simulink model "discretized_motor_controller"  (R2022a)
settings: Solver=VariableStepAuto  StartTime=0.0  StopTime=10  RelTol=1e-3
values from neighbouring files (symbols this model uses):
  B = 1e-5    (= 1e-05)    [motor_controller.m]
  J = 1e-4    (= 0.0001)    [motor_controller.m]
  k = 2e-2    (= 0.02)    [motor_controller.m]
  Ka_i = 1 / Kp_i    (= 0.2)    [motor_controller.m]
  Ka_s = 1 / Kp_s    (= 0.2)    [motor_controller.m]
  Ki_i = Kp_i * Ra / La    (= 1000)    [motor_controller.m]
  Ki_s = J * omega_cs^2 / (5 * k)    (= 1000)    [motor_controller.m]
  Kp_i = La * omega_cc    (= 5)    [motor_controller.m]
  Kp_p = 2.5    [motor_controller.m]
  Kp_s = J * omega_cs / k    (= 5)    [motor_controller.m]
  La = 1e-3    (= 0.001)    [motor_controller.m]
  Ra = 0.2    [motor_controller.m]
  T_sample = 1 / f_sample    (= 1e-05)    [motor_controller.m]
undefined symbols (not defined in the file or in its folder): DiscIntNeverNeededParam

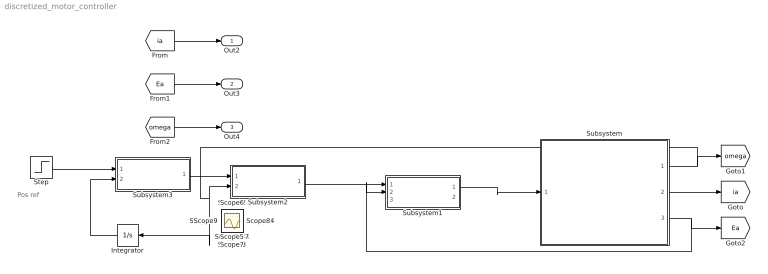
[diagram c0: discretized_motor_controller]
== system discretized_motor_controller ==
  note: Pos ref
  Integrator : Integrator
  Step : Step  After=180  SampleTime=0
  Subsystem : Subsystem  Tag=PMDC  Description=PMDC
  Subsystem1 : Subsystem  Description=PI controller
  Subsystem2 : Subsystem  Description=PI controller
  Subsystem3 : Subsystem  Description=PI controller
  Out2 : Outport
  Out3 : Outport  Port=2
  Out4 : Outport  Port=3
  Scope{,1..34} (35 alike) : Scope
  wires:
  Subsystem/1(Out1) -> Subsystem2/2(In4), Integrator/1, [omega]
  [ia] -> Out2/1
  [Ea] -> Out3/1
  [omega] -> Out4/1
  Subsystem/3(Out3) -> Subsystem1/2(In2), [Ea]
  Subsystem/2(Out2) -> [ia]
  Step/1 -> Subsystem3/1(In1)
  Integrator/1 -> Subsystem3/2(In3)
  Subsystem3/1(Out1) -> Subsystem2/1(In1)
  Subsystem1/1(Out1) -> Subsystem/1(In1)
  Subsystem2/1(Out2) -> Subsystem1/1(In1)

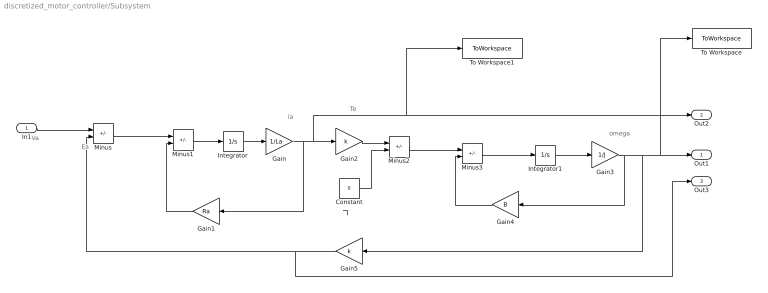
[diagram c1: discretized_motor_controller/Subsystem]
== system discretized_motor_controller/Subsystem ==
  note: Ea
  note: Va
  note: Te
  note: Tl
  note: omega
  note: ia
  In1 : Inport
  Constant : Constant  Value=0
  Gain : Gain  Gain=1/La
  Gain1 : Gain  Gain=Ra
  Gain2 : Gain  Gain=k
  Gain3 : Gain  Gain=1/J
  Gain4 : Gain  Gain=B
  Gain5 : Gain  Gain=k
  Integrator : Integrator
  Integrator1 : Integrator
  Minus{,1..3} (4 alike) : Sum  Inputs=+-
  To Workspace : ToWorkspace  VariableName=omega_simout  SaveFormat=Timeseries  SampleTime=-1
  To Workspace1 : ToWorkspace  VariableName=current_simout  SaveFormat=Timeseries  SampleTime=-1
  Out1 : Outport
  Out2 : Outport  Port=2
  Out3 : Outport  Port=3
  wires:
  Minus/1 -> Minus1/1
  Gain1/1 -> Minus1/2
  Minus1/1 -> Integrator/1
  Integrator/1 -> Gain/1
  Gain/1 -> To Workspace1/1, Out2/1, Gain2/1, Gain1/1
  Gain2/1 -> Minus2/1
  Constant/1 -> Minus2/2
  Minus2/1 -> Minus3/1
  Minus3/1 -> Integrator1/1
  Integrator1/1 -> Gain3/1
  Gain4/1 -> Minus3/2
  In1/1 -> Minus/1
  Gain5/1 -> Out3/1, Minus/2
  Gain3/1 -> Gain4/1, Gain5/1, To Workspace/1, Out1/1

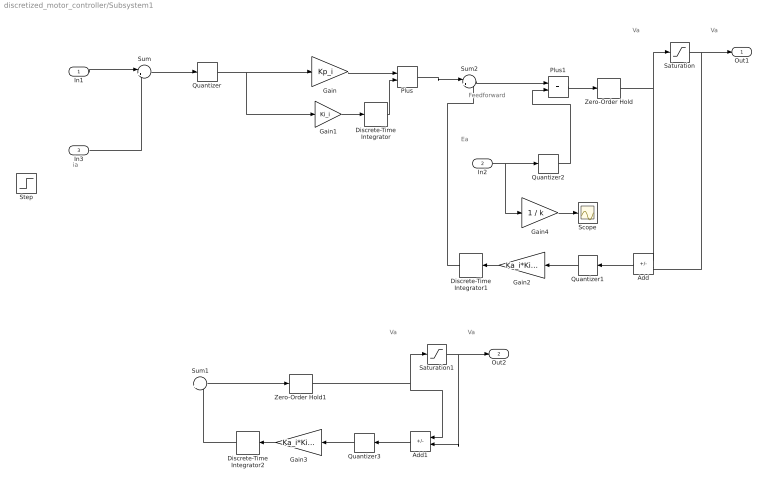
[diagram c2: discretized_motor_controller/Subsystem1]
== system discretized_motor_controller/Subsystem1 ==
  note: ia
  note: Ea
  note: Feedforward
  note: Va
  note: Va
  note: Va
  note: Va
  In1 : Inport
  In2 : Inport  Port=2
  In3 : Inport  Port=3
  Add : Sum  Inputs=+-
  Add1 : Sum  Inputs=+-
  Discrete-Time Integrator : DiscreteIntegrator  SampleTime=T_sample  ICPrevOutput=DiscIntNeverNeededParam  ICPrevScaledInput=DiscIntNeverNeededParam
  Discrete-Time Integrator1 : DiscreteIntegrator  SampleTime=T_sample  ICPrevOutput=DiscIntNeverNeededParam  ICPrevScaledInput=DiscIntNeverNeededParam
  Discrete-Time Integrator2 : DiscreteIntegrator  SampleTime=T_sample  ICPrevOutput=DiscIntNeverNeededParam  ICPrevScaledInput=DiscIntNeverNeededParam
  Gain : Gain  Gain=Kp_i
  Gain1 : Gain  Gain=Ki_i
  Gain2 : Gain  Gain=Ka_i*Ki_i
  Gain3 : Gain  Gain=Ka_i*Ki_i
  Gain4 : Gain  Gain=1 / k
  Plus : Sum
  Plus1 : Sum
  Quantizer{,1..3} (4 alike) : Quantizer  QuantizationInterval=T_sample
  Saturation : Saturate  UpperLimit=12  LowerLimit=-12
  Saturation1 : Saturate  UpperLimit=12  LowerLimit=-12
  Scope : Scope
  Step : Step  Before=1  SampleTime=0
  Sum : Sum  Inputs=|+-
  Sum1 : Sum  Inputs=|+-
  Sum2 : Sum  Inputs=|+-
  Zero-Order Hold : ZeroOrderHold  SampleTime=T_sample
  Zero-Order Hold1 : ZeroOrderHold  SampleTime=T_sample
  Out1 : Outport
  Out2 : Outport  Port=2
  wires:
  Gain1/1 -> Discrete-Time Integrator/1
  In1/1 -> Sum/1
  Gain/1 -> Plus/1
  Discrete-Time Integrator/1 -> Plus/2
  Quantizer2/1 -> Plus1/2
  Plus1/1 -> Zero-Order Hold/1
  Saturation/1 -> Add/2, Out1/1
  In3/1 -> Sum/2
  Gain2/1 -> Discrete-Time Integrator1/1
  Discrete-Time Integrator1/1 -> Sum2/2
  Sum2/1 -> Plus1/1
  Quantizer/1 -> Gain1/1, Gain/1
  Quantizer1/1 -> Gain2/1
  Add/1 -> Quantizer1/1
  In2/1 -> Gain4/1, Quantizer2/1
  Zero-Order Hold/1 -> Add/1, Saturation/1
  Sum/1 -> Quantizer/1
  Gain3/1 -> Discrete-Time Integrator2/1
  Discrete-Time Integrator2/1 -> Sum1/2
  Quantizer3/1 -> Gain3/1
  Saturation1/1 -> Add1/2, Out2/1
  Sum1/1 -> Zero-Order Hold1/1
  Add1/1 -> Quantizer3/1
  Zero-Order Hold1/1 -> Add1/1, Saturation1/1
  Plus/1 -> Sum2/1
  Gain4/1 -> Scope/1

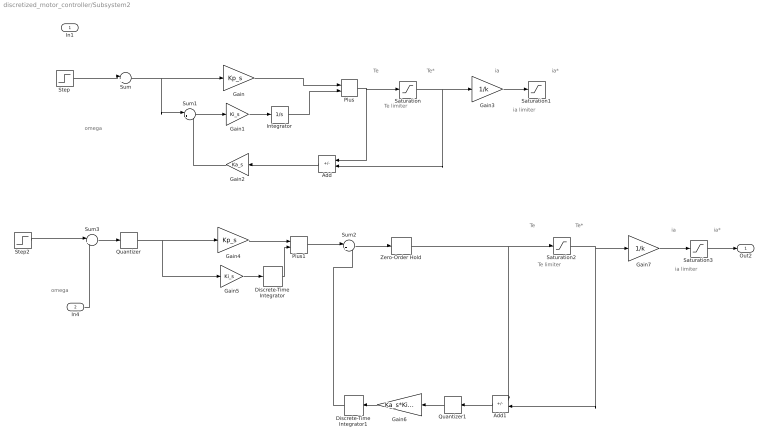
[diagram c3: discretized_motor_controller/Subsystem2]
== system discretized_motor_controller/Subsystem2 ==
  note: omega
  note: Te
  note: ia
  note: Te limiter
  note: Te*
  note: ia*
  note: ia limiter
  note: Te
  note: Te*
  note: Te limiter
  note: ia
  note: ia*
  note: ia limiter
  note: omega
  In1 : Inport
  In4 : Inport  Port=2
  Add : Sum  Inputs=+-
  Add1 : Sum  Inputs=+-
  Discrete-Time Integrator : DiscreteIntegrator  SampleTime=T_sample  ICPrevOutput=DiscIntNeverNeededParam  ICPrevScaledInput=DiscIntNeverNeededParam
  Discrete-Time Integrator1 : DiscreteIntegrator  SampleTime=T_sample  ICPrevOutput=DiscIntNeverNeededParam  ICPrevScaledInput=DiscIntNeverNeededParam
  Gain : Gain  Gain=Kp_s
  Gain1 : Gain  Gain=Ki_s
  Gain2 : Gain  Gain=Ka_s
  Gain3 : Gain  Gain=1/k
  Gain4 : Gain  Gain=Kp_s
  Gain5 : Gain  Gain=Ki_s
  Gain6 : Gain  Gain=Ka_s*Ki_s
  Gain7 : Gain  Gain=1/k
  Integrator : Integrator
  Plus : Sum
  Plus1 : Sum
  Quantizer : Quantizer  QuantizationInterval=T_sample
  Quantizer1 : Quantizer  QuantizationInterval=T_sample
  Saturation : Saturate  UpperLimit=0.247  LowerLimit=-0.247
  Saturation1 : Saturate  UpperLimit=1  LowerLimit=-1
  Saturation2 : Saturate  UpperLimit=0.247  LowerLimit=-0.247
  Saturation3 : Saturate  UpperLimit=1  LowerLimit=-1
  Step : Step  Time=0  After=597  SampleTime=0
  Step2 : Step  After=300  SampleTime=0
  Sum{,1..3} (4 alike) : Sum  Inputs=|+-
  Zero-Order Hold : ZeroOrderHold  SampleTime=T_sample
  Out2 : Outport
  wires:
  Gain1/1 -> Integrator/1
  Sum/1 -> Sum1/1, Gain/1
  Gain/1 -> Plus/1
  Integrator/1 -> Plus/2
  Plus/1 -> Saturation/1, Add/1
  Saturation/1 -> Gain3/1, Add/2
  Sum1/1 -> Gain1/1
  Gain2/1 -> Sum1/2
  ? -> Sum/2
  Add/1 -> Gain2/1
  Gain3/1 -> Saturation1/1
  Step/1 -> Sum/1
  Sum2/1 -> Zero-Order Hold/1
  Gain4/1 -> Plus1/1
  Discrete-Time Integrator/1 -> Plus1/2
  Quantizer/1 -> Gain5/1, Gain4/1
  Plus1/1 -> Sum2/1
  Gain5/1 -> Discrete-Time Integrator/1
  Saturation2/1 -> Gain7/1, Add1/2
  Add1/1 -> Quantizer1/1
  Discrete-Time Integrator1/1 -> Sum2/2
  Quantizer1/1 -> Gain6/1
  Gain6/1 -> Discrete-Time Integrator1/1
  Zero-Order Hold/1 -> Add1/1, Saturation2/1
  Gain7/1 -> Saturation3/1
  Saturation3/1 -> Out2/1
  Saturation1/1 -> ?
  In4/1 -> Sum3/2
  Sum3/1 -> Quantizer/1
  Step2/1 -> Sum3/1

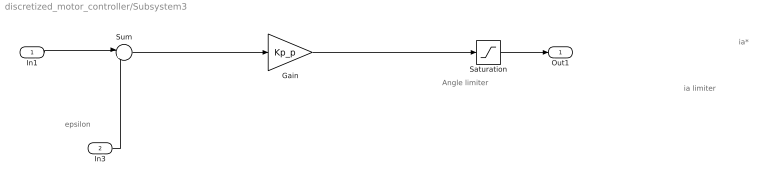
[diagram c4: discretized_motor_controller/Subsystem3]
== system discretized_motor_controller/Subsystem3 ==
  note: epsilon
  note: Angle limiter
  note: ia*
  note: ia limiter
  In1 : Inport
  In3 : Inport  Port=2
  Gain : Gain  Gain=Kp_p
  Saturation : Saturate  UpperLimit=360  LowerLimit=0
  Sum : Sum  Inputs=|+-
  Out1 : Outport
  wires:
  Sum/1 -> Gain/1
  In1/1 -> Sum/1
  In3/1 -> Sum/2
  Saturation/1 -> Out1/1
  Gain/1 -> Saturation/1
